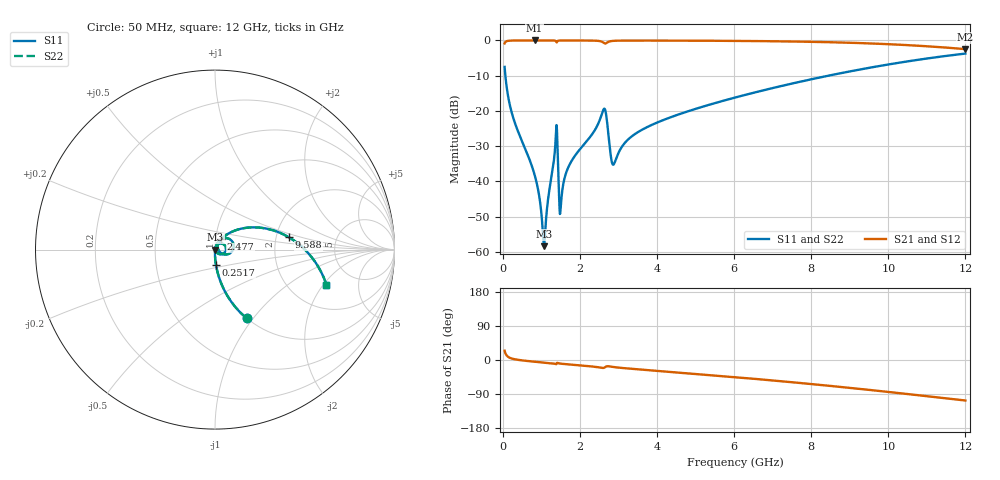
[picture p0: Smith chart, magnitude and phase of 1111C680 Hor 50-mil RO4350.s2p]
# GHz S MA R 50
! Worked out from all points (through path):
!   1601 points, 50 MHz to 12 GHz, reference 50 ohm
!   highest |S21| = -0.01 dB at 826.8 MHz (marker M1); lowest = -2.5 dB at 12 GHz (marker M2)
!   group delay of S21, straight-line fit = 25 ps
!   lowest |S11| = -58.4 dB at 1.073 GHz (marker M3), VSWR 1.00, Z = 50.1 - j0.0101 ohm
!   |S11| at or under -10 dB: 69.65 MHz to 8.448 GHz (8.379 GHz wide, 197 % of centre)
!   |S22| runs from -58.4 to -3.7 dB; largest |S21 - S12| = 0
!   S11 on the Smith chart (normalised r, x): 50 MHz: 1.00, -0.93; 251.7 MHz: 1.00, -0.18; 2.477 GHz: 1.06, +0.12; 9.588 GHz: 2.35, +0.39; 12 GHz: 3.17, -2.14
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0.05  0.4214 -65.3  0.9065 24.6  0.9065 24.6  0.4214 -65.3
0.2516563  0.0876 -86.2  0.9955 3.4  0.9955 3.4  0.0876 -86.2
0.82675  0.01246 -89.9  0.9989 -4.5  0.9989 -4.5  0.01246 -89.9
0.9313125  0.006993 -86.6  0.9988 -5.5  0.9988 -5.5  0.006993 -86.6
1.073219  0.001206 -4.8  0.9987 -6.7  0.9987 -6.7  0.001206 -4.8
1.3645  0.03282 60.5  0.9887 -10.3  0.9887 -10.3  0.03282 60.5
1.401844  0.06215 -8.1  0.9378 -8.8  0.9378 -8.8  0.06215 -8.1
1.476531  0.003897 -21.1  0.9961 -9.2  0.9961 -9.2  0.003897 -21.1
1.513875  0.00497 49.8  0.9974 -9.7  0.9974 -9.7  0.00497 49.8
1.685656  0.01515 72.2  0.9981 -11.4  0.9981 -11.4  0.01515 72.2
2.044156  0.03042 71.4  0.9973 -14.5  0.9973 -14.5  0.03042 71.4
2.477344  0.06589 60.1  0.9854 -19.2  0.9854 -19.2  0.06589 60.1
2.649125  0.1061 9.1  0.9053 -19.4  0.9053 -19.4  0.1061 9.1
2.813438  0.02122 -13.3  0.9787 -17.6  0.9787 -17.6  0.02122 -13.3
2.880656  0.01749 24.4  0.987 -18.6  0.987 -18.6  0.01749 24.4
3.269031  0.0401 61.6  0.995 -22.6  0.995 -22.6  0.0401 61.6
4.038312  0.0696 58.8  0.9945 -28.9  0.9945 -28.9  0.0696 58.8
6.025  0.1547 43.5  0.9845 -45.3  0.9845 -45.3  0.1547 43.5
8.019156  0.2822 25.6  0.9549 -63.6  0.9549 -63.6  0.2822 25.6
9.587594  0.4165 9.6  0.9038 -79.8  0.9038 -79.8  0.4165 9.6
10.01331  0.4569 5.0  0.8839 -84.4  0.8839 -84.4  0.4569 5.0
12  0.6506 -17.4  0.7527 -106.9  0.7527 -106.9  0.6506 -17.4
